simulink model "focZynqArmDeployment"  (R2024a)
settings: Solver=ode45  StartTime=0.0  StopTime=10.0  RelTol=1e-3  EnableMultiTasking=on
StartFcn:
  | demo.externalMode.deleteLoggedData(bdroot);
StopFcn:
  | demo.externalMode.loadLoggedDataIntoSdi(bdroot);
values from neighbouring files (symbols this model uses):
  commandTypeEnum = Error
                        0
                        Command: Error
                    
                    
                        OpenLoopVelocity
                        1
                        Command: Open-loop velocity control
                    
                    
                        CalibrateEncoder
                        2
                        Command: Calibrate encoder    [focZynqData.sldd]
  inputSourceEnum = StandAloneTest
                        0
                        Type: Stand alone
                    
                    
                        InteractiveUserInput
                        1
                        Type: Interactive
                    
                
                Input type enumeration
                
                
                StandAloneTest    [focZynqData.sldd]
libraries: simulink x3, focZynqHdlAxiInterfaceLib x1, SignalEditorBlockLib x1

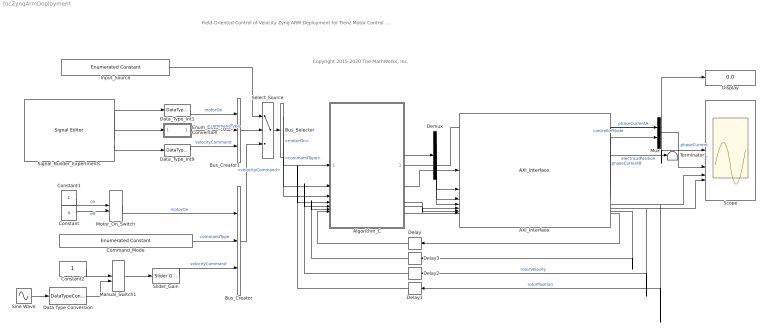
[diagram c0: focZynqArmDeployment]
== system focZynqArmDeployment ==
  note: Field-Oriented Control of Velocity Zynq ARM Deployment for Trenz Motor Control Kit
  note: Copyright 2015-2020 The MathWorks, Inc.
  AXI_Interface : focZynqHdlAxiInterfaceLib/AXI_Interface
  Algorithm_C : ModelReference  ModelNameDialog=focZynqC  SimulationMode=Normal  ModelReferenceVersion=8.2
  Bus_Creator : BusCreator  Inputs=3
  Bus_Creator1 : BusCreator  Inputs=3
  Bus_Selector : BusSelector  OutputSignals=motorOn,commandType,velocityCommand
  Command_Mode : simulink/Sources/Enumerated Constant  OutDataTypeStr=Enum: commandTypeEnum  Value=commandTypeEnum.Velocity  SampleTime=-1
  Constant : Constant  Value=0  OutDataTypeStr=boolean  SampleTime=-1
  Constant1 : Constant  OutDataTypeStr=boolean  SampleTime=-1
  Constant2 : Constant  OutDataTypeStr=single  SampleTime=-1
  Data Type Conversion : DataTypeConversion  OutDataTypeStr=single
  Data_Type_Int1 : DataTypeConversion  OutDataTypeStr=boolean
  Data_Type_Int9 : DataTypeConversion  OutDataTypeStr=single
  Delay{,1..3} (4 alike) : Delay  DelayLength=1
  Demux : Demux  Outputs=3
  Display : Display
  Enum_Data_Type_Conversion : Subsystem  mask(Convert to enumerated data type){dataTypeStr=Enum: commandTypeEnum}
      mask prompts: dataTypeStr "Output data type"
  Input_Source : simulink/Sources/Enumerated Constant  OutDataTypeStr=Enum: inputSourceEnum  Value=inputSourceEnum.StandAloneTest  SampleTime=-1
  Manual_Switch1 : ManualSwitch
  Motor_On_Switch : ManualSwitch  CurrentSetting=0
  Mux : Mux  Inputs=2
  Scope : Scope  NumInputPorts=4
  Select_Source : MultiPortSwitch  DataPortOrder=Specify indices  DataPortIndices={inputSourceEnum.StandAloneTest, inputSourceEnum.InteractiveUserInput}  DiagnosticForDefault=None
  Signal_Builder_Experiments : SignalEditorBlockLib/Signal Editor  FileName=ARMModelInputs.mat  ActiveScenario=Calibrate_Velocity_steps  ActiveSignal=velocityCommand (rad/sec)  IsBus=off  OutputBusObjectStr=Bus: BusObject  SampleTime=-1  ZeroCross=off  OutputAfterFinalValue=Extrapolation  Unit=inherit  PreserveSignalName=on  ApplySigPropsToAllScenarios=on  ApplySigPropsToAllSignals=off
  Sine Wave : Sin  Frequency=0.5*2*pi  SampleTime=1e-3
  Slider_Gain : simulink/Math Operations/Slider Gain  gain=100  low=-400  high=400
  Terminator1 : Terminator
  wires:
  Constant/1 -> Motor_On_Switch/2  "off"
  Constant1/1 -> Motor_On_Switch/1  "on"
  Constant2/1 -> Manual_Switch1/1
  Data Type Conversion/1 -> Manual_Switch1/2
  Manual_Switch1/1 -> Slider_Gain/1
  Bus_Selector/1 -> Algorithm_C/1  "<motorOn>"
  Bus_Selector/2 -> Algorithm_C/2  "<commandType>"
  Bus_Selector/3 -> Algorithm_C/3  "<velocityCommand>"
  Bus_Creator1/1 -> Select_Source/2
  Input_Source/1 -> Select_Source/1
  Motor_On_Switch/1 -> Bus_Creator/1  "motorOn"
  Command_Mode/1 -> Bus_Creator/2  "commandType"
  Bus_Creator/1 -> Select_Source/3
  Select_Source/1 -> Bus_Selector/1
  Data_Type_Int1/1 -> Bus_Creator1/1  "motorOn"
  Signal_Builder_Experiments/2 -> Enum_Data_Type_Conversion/1(In)
  Data_Type_Int9/1 -> Bus_Creator1/3  "velocityCommand"
  Enum_Data_Type_Conversion/1(Out) -> Bus_Creator1/2  "commandType"
  AXI_Interface/7 -> Delay/1
  AXI_Interface/4 -> Delay1/1, Scope/3  "rotorPosition"
  AXI_Interface/5 -> Delay2/1, Scope/4  "rotorVelocity"
  AXI_Interface/6 -> Delay3/1
  Signal_Builder_Experiments/1 -> Data_Type_Int1/1
  Signal_Builder_Experiments/3 -> Data_Type_Int9/1
  Slider_Gain/1 -> Bus_Creator/3  "velocityCommand"
  Delay2/1 -> Algorithm_C/5
  Delay3/1 -> Algorithm_C/6
  Delay1/1 -> Algorithm_C/4
  Delay/1 -> Algorithm_C/7
  AXI_Interface/2 -> Mux/2  "phaseCurrentB"
  AXI_Interface/1 -> Mux/1  "phaseCurrentA"
  AXI_Interface/3 -> Terminator1/1  "electricalPosition"
  Algorithm_C/1 -> Scope/1, Display/1  "controllerMode"
  Demux/2 -> AXI_Interface/3
  Demux/1 -> AXI_Interface/2
  Demux/3 -> AXI_Interface/4
  Algorithm_C/3 -> Demux/1
  Algorithm_C/2 -> AXI_Interface/1
  Algorithm_C/4 -> AXI_Interface/5
  Algorithm_C/5 -> AXI_Interface/6
  Algorithm_C/6 -> AXI_Interface/7
  Mux/1 -> Scope/2  "phaseCurrent"
  Sine Wave/1 -> Data Type Conversion/1

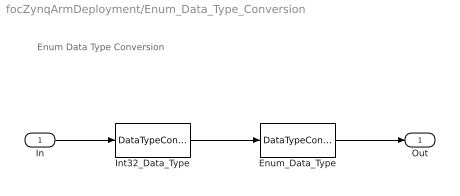
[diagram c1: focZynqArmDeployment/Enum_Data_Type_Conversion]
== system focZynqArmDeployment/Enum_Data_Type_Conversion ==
  note: Enum Data Type Conversion
  In : Inport
  Enum_Data_Type : DataTypeConversion  OutDataTypeStr=dataTypeStr
  Int32_Data_Type : DataTypeConversion  OutDataTypeStr=int32
  Out : Outport
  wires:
  In/1 -> Int32_Data_Type/1
  Int32_Data_Type/1 -> Enum_Data_Type/1
  Enum_Data_Type/1 -> Out/1
